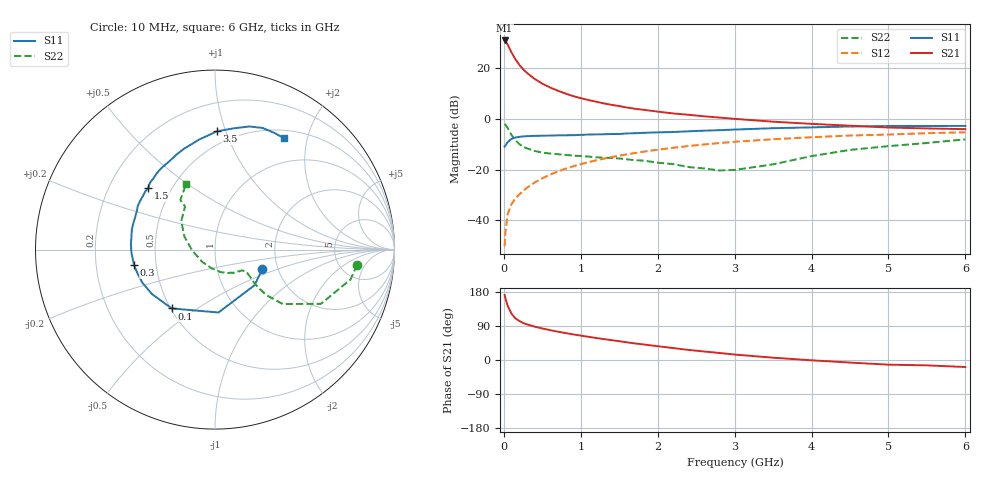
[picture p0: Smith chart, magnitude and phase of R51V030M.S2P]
! SIEMENS Small Signal Semiconductors
! BFR183
! Si NPN RF Bipolar Junction Transistor in SOT23
! VCE = 1 V  IC = 30 mA
! Common Emitter S-Parameters:  May  1996
# GHz  S  MA  R  50
!  f  S11  S21  S12  S22
! GHz  MAG  ANG  MAG  ANG  MAG  ANG  MAG  ANG
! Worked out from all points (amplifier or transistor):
!   36 points, 10 MHz to 6 GHz, reference 50 ohm
!   highest |S21| = 31.0 dB at 10 MHz (marker M1)
!   |S21| within 3 dB of that: start of sweep to 71.7 MHz
!   unconditionally stable (mu >= 1): start of sweep to 17.87 MHz; 210.7 MHz to 4.447 GHz; 4.541 GHz to end of sweep
!   at 250 MHz: K = 1.05, MAG = 22.7 dB, |S12| = -28.3 dB
!   at 1.4 GHz: K = 1.16, MAG = 7.9 dB, |S12| = -15.0 dB
!   at 6 GHz: K = 1.03, MAG = -0.4 dB, |S12| = -5.2 dB
!   S11 on the Smith chart (normalised r, x): 10 MHz: 1.66, -0.39; 100 MHz: 0.51, -0.40; 300 MHz: 0.37, -0.08; 1.5 GHz: 0.37, +0.34; 3.5 GHz: 0.40, +0.93; 6 GHz: 0.61, +1.63
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0.01  0.2853 -22.3  35.51 171.4  0.0031 76.3  0.7962 -6.1
0.02  0.2966 -42.0  34.66 163.2  0.0059 73.3  0.7736 -12.4
0.05  0.3509 -86.8  29.33 142.8  0.0134 67.0  0.6632 -27.1
0.1  0.4069 -126.3  20.56 122.0  0.0209 62.9  0.484 -38.8
0.15  0.4304 -145.1  15.14 110.1  0.0273 62.8  0.3831 -41.5
0.2  0.4454 -155.9  11.83 103.0  0.0324 64.3  0.3217 -41.3
0.25  0.4527 -163.8  9.631 97.8  0.0383 65.9  0.2845 -40.3
0.3  0.4592 -169.3  8.148 94.0  0.0439 67.8  0.2638 -38.9
0.4  0.4658 -177.8  6.197 88.1  0.056 69.3  0.2351 -36.9
0.5  0.4692 176.7  4.979 83.2  0.0677 70.3  0.217 -35.6
0.6  0.471 171.4  4.195 78.8  0.0796 70.3  0.2087 -35.5
0.8  0.478 162.0  3.185 71.2  0.1043 69.0  0.1964 -36.7
0.9  0.4799 158.0  2.838 67.6  0.1165 68.5  0.1899 -37.7
1.1  0.4943 150.5  2.37 61.2  0.1408 66.8  0.1815 -42.0
1.5  0.5063 137.3  1.801 49.6  0.189 61.9  0.1667 -50.8
1.7  0.5248 130.7  1.598 43.8  0.2128 59.3  0.1545 -56.2
2.2  0.5546 117.1  1.29 31.5  0.2705 52.3  0.1291 -76.4
2.8  0.6026 102.3  1.07 18.6  0.3357 43.3  0.0967 -118.7
3.5  0.6594 89.0  0.886 6.1  0.3991 32.4  0.1277 -178.3
4.5  0.7123 74.4  0.739 -6.8  0.4727 18.2  0.246 139.8
5.5  0.7295 63.0  0.652 -14.2  0.5254 6.5  0.337 124.9
6  0.7302 58.0  0.632 -18.5  0.5471 -1.1  0.3975 114.1
